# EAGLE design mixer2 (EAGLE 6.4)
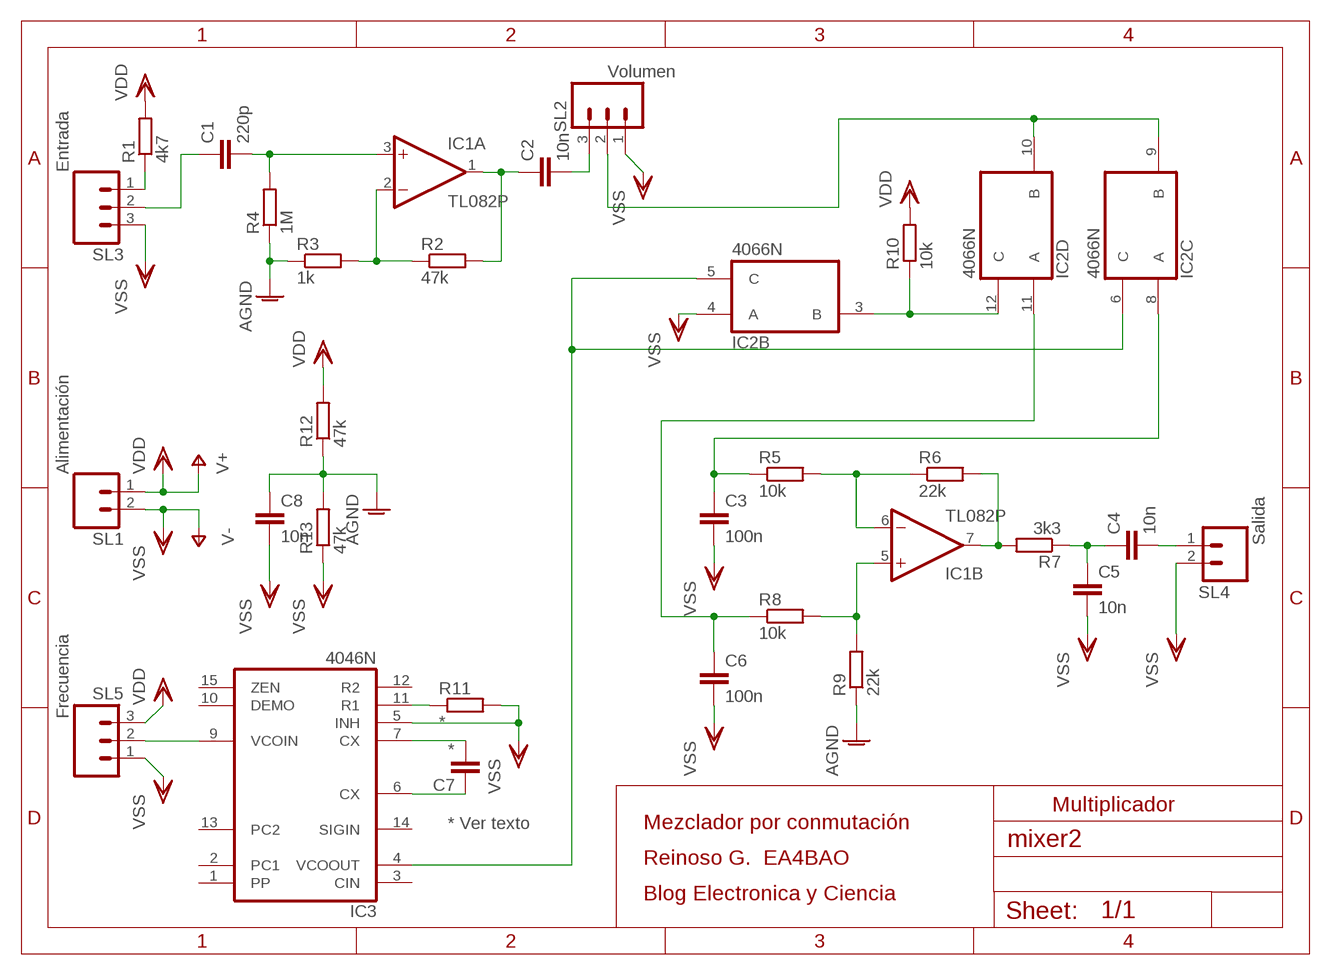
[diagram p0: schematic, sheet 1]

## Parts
C1  220p  C-EU050-035X075  [C050-035X075]
C2  10n  C-EU050-035X075  [C050-035X075]
C3  100n  C-EU050-035X075  [C050-035X075]
C4  10n  C-EU050-035X075  [C050-035X075]
C5  10n  C-EU050-035X075  [C050-035X075]
C6  100n  C-EU050-035X075  [C050-035X075]
C7  *  C-EU050-035X075  [C050-035X075]
C8  10n  C-EU050-035X075  [C050-035X075]
IC1  TL082P  [DIL08]
IC2  4066N  [DIL14]
IC3  4046N  [DIL16]
R1  4k7  R-EU_0207/10  [0207/10]
R2  47k  R-EU_0207/10  [0207/10]
R3  1k  R-EU_0207/10  [0207/10]
R4  1M  R-EU_0207/10  [0207/10]
R5  10k  R-EU_0207/10  [0207/10]
R6  22k  R-EU_0207/10  [0207/10]
R7  3k3  R-EU_0207/10  [0207/10]
R8  10k  R-EU_0207/10  [0207/10]
R9  22k  R-EU_0207/10  [0207/10]
R10  10k  R-EU_0207/10  [0207/10]
R11  *  R-EU_0207/10  [0207/10]
R12  47k  R-EU_0207/10  [0207/10]
R13  47k  R-EU_0207/10  [0207/10]
SL1  Alimentación  M02  [02P]
SL2  Volumen  M03  [03P]
SL3  Entrada  M03  [03P]
SL4  Salida  M02  [02P]
SL5  Frecuencia  M03  [03P]

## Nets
AGND: C8.1 R3.1 R4.1 R9.1 R12.1 R13.2
FLOC: IC2.5(B:C) IC2.6(C:C) IC3.4(VCOOUT)
N$1: R1.1 SL3.1
N$2: C1.1 SL3.2
N$3: C1.2 IC1.3(A:+IN) R4.2
N$4: IC1.6(B:-IN) R5.2 R6.1
N$5: IC1.2(A:-IN) R2.1 R3.2
N$6: C4.1 C5.1 R7.1
N$7: C2.1 IC1.1(A:OUT) R2.2
N$8: C4.2 SL4.1
N$9: C2.2 SL2.3
N$11: IC2.3(B:B) IC2.12(D:C) R10.1
N$12: IC2.9(C:B) IC2.10(D:B) SL2.2
N$13: IC3.9(VCOIN) SL5.2
N$14: IC3.11(R1) R11.1
N$15: C7.1 IC3.6(CX)
N$16: C7.2 IC3.7(CX)
N$18: IC1.7(B:OUT) R6.2 R7.2
N$20: C3.1 IC2.8(C:A) R5.1
N$21: C6.1 IC2.11(D:A) R8.1
N$23: IC1.5(B:+IN) R8.2 R9.2
VDD: R1.2 R10.2 R12.2 SL1.1 SL5.3 ; supply symbol labelled V+
VSS: C3.2 C5.2 C6.2 C8.2 IC2.4(B:A) IC3.5(INH) R11.2 R13.1 SL1.2 SL2.1 SL3.3 SL4.2 SL5.1 ; supply symbol labelled V-
Unconnected: IC2.1(A:A) IC2.2(A:B) IC2.13(A:C) IC3.1(PP) IC3.2(PC1) IC3.3(CIN) IC3.10(DEMO) IC3.12(R2) IC3.13(PC2) IC3.14(SIGIN) IC3.15(ZEN)

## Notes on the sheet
- Multiplicador
- * Ver texto | Mezclador por conmutación
- Reinoso G.  EA4BAO
- Blog Electronica y Ciencia

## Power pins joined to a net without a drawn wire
VDD: IC1.8(P:V+) IC2.14(P:VDD) IC3.16(VDD)
VSS: IC1.4(P:V-) IC2.7(P:VSS) IC3.8(VSS)

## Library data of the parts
C1-C8 = rcl:C-EU: CAPACITOR, European symbol
IC1 = linear:TL082: OP AMP
IC2 = 40xx:4066: Quad bilateral ANALOG SWITCH
IC3 = 40xx:4046: Micropower PLL
R1-R13 = rcl:R-EU_: RESISTOR, European symbol
SL1 SL4 = con-amp-quick:M02: AMP QUICK CONNECTOR; OC_FARNELL: unknown; OC_NEWARK: unknown
SL2 SL3 SL5 = con-amp-quick:M03: AMP QUICK CONNECTOR; OC_FARNELL: unknown; OC_NEWARK: unknown

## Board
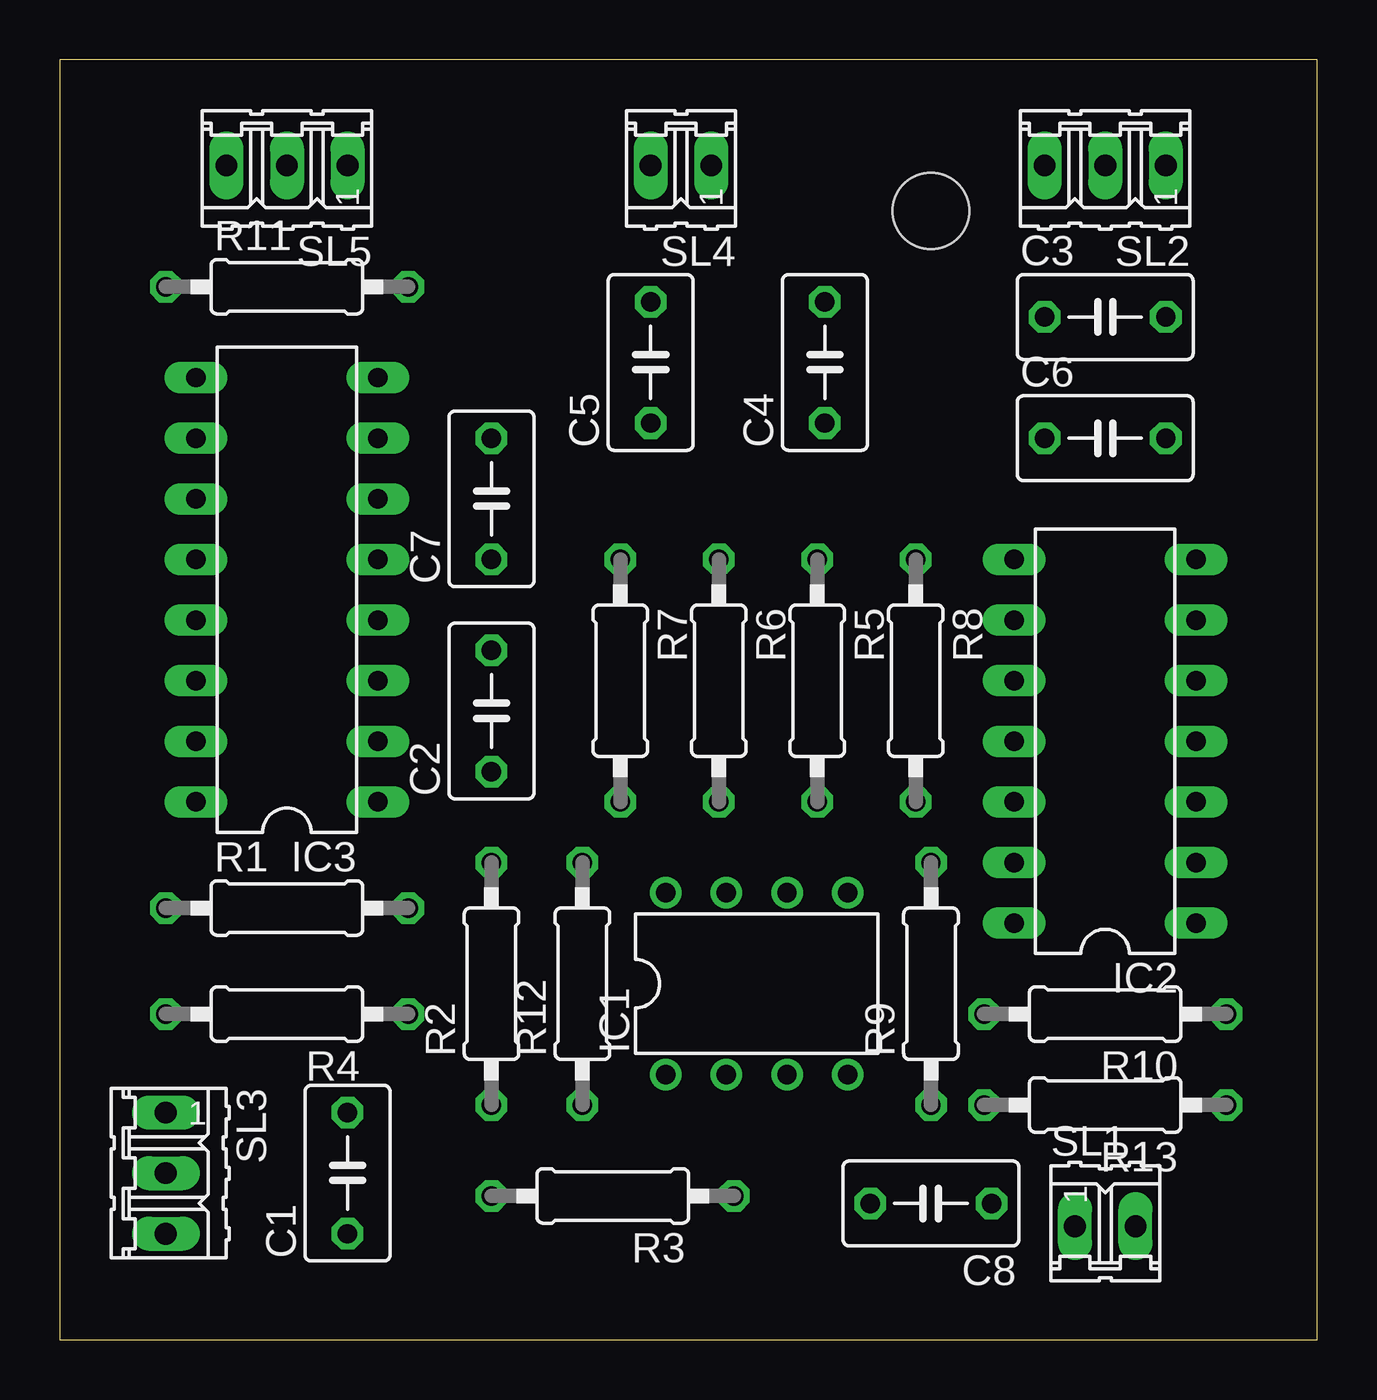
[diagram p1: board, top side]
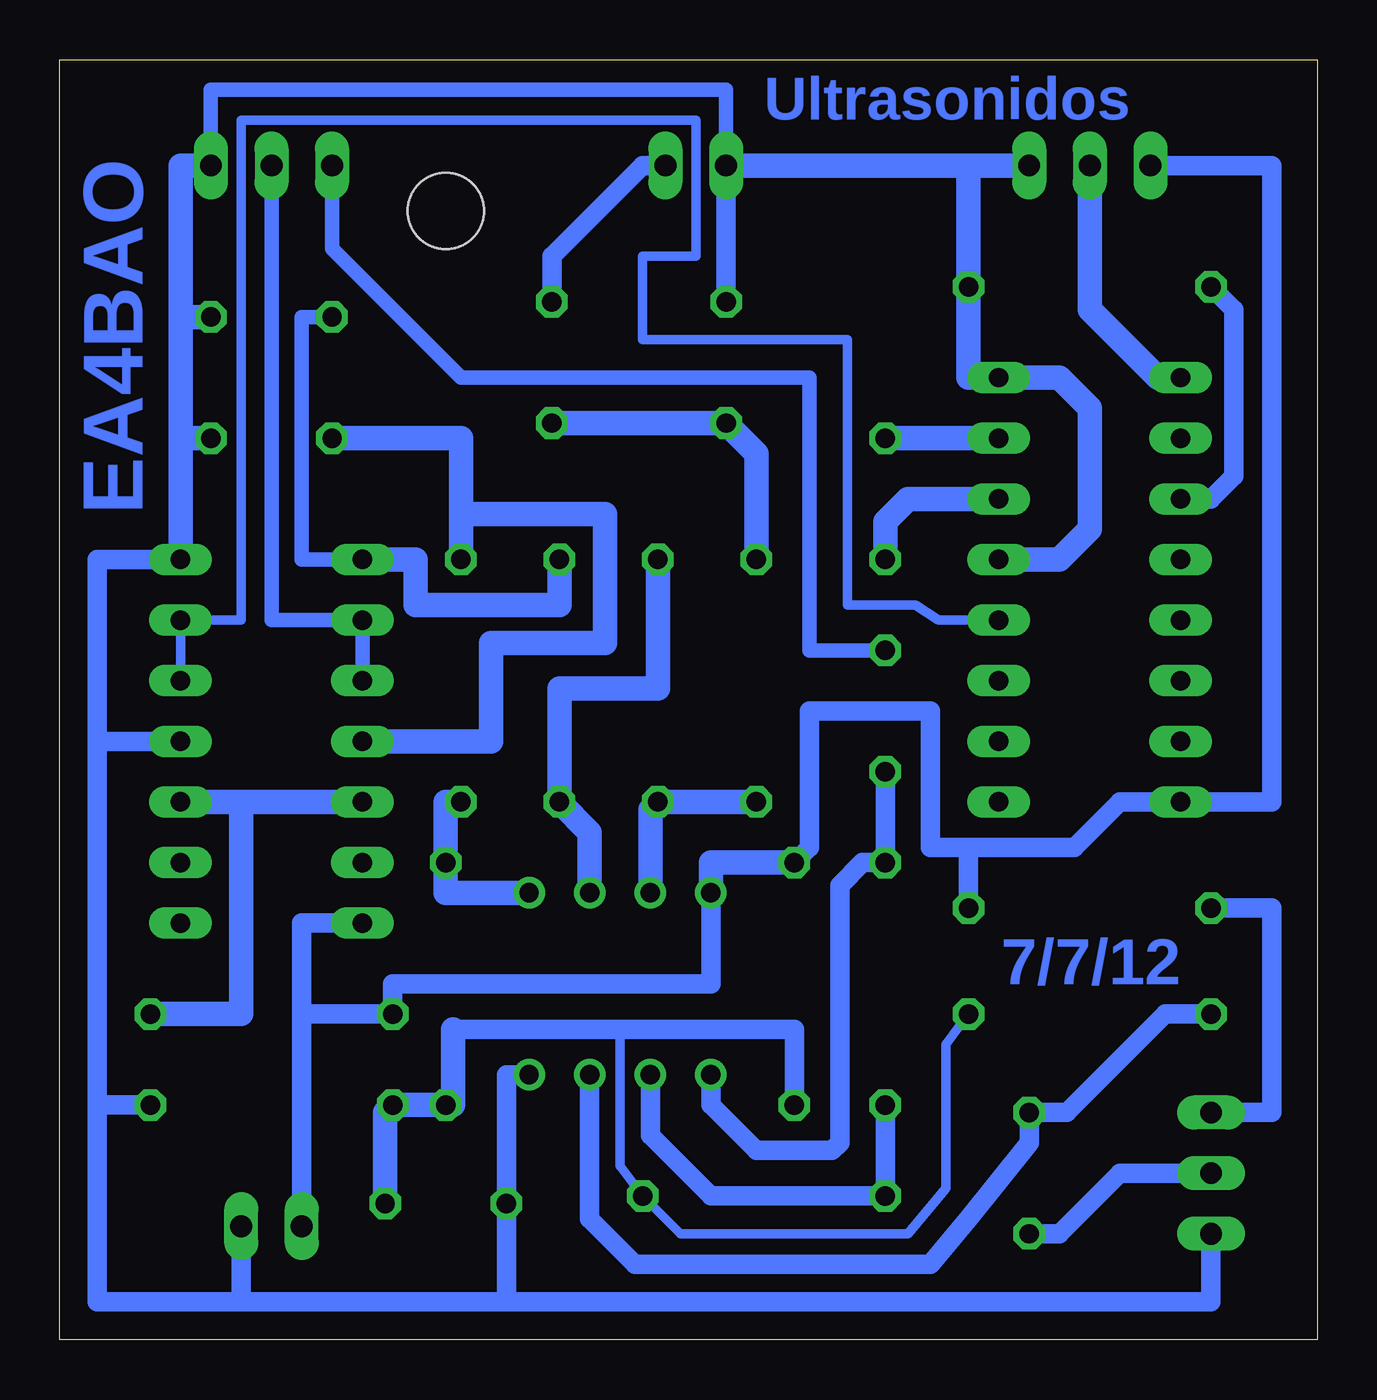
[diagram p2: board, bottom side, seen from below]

Size 52.69 x 53.65 mm. Coordinates in mm from the lower left corner, seen from the top.
Outline: 0,0 52.69,0 52.69,53.65 0,53.65 0,0
Copper layers (1*16): Top 0.035mm / dielectric 1.5mm / Bottom 0.035mm
Design rules "default": minimum track width 10mil, minimum drill 24mil, track to track 8mil, track to pad 8mil, pad to pad 8mil, via to via 8mil, smd to smd 8mil, copper to edge 40mil, drill to drill 8mil, minimum pad ring 10mil, minimum via ring 8mil, stop-mask expansion 4mil, vias tented up to drill 0mil, thermal gap 10mil
Holes 3.2 mm at 36.51,47.31

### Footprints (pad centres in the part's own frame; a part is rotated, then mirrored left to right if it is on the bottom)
C050-035X075 = drill 0.813 octagon: 1 -2.54,0; 2 2.54,0
DIL08 = drill 0.813 pad 1.27: 1 -3.81,-3.81; 2 -1.27,-3.81; 3 1.27,-3.81; 4 3.81,-3.81; 5 3.81,3.81; 6 1.27,3.81; 7 -1.27,3.81; 8 -3.81,3.81
DIL14 = drill 0.813 long: 1 -7.62,-3.81; 2 -5.08,-3.81; 3 -2.54,-3.81; 4 0,-3.81; 5 2.54,-3.81; 6 5.08,-3.81; 7 7.62,-3.81; 8 7.62,3.81; 9 5.08,3.81; 10 2.54,3.81; 11 0,3.81; 12 -2.54,3.81; 13 -5.08,3.81; 14 -7.62,3.81
DIL16 = drill 0.813 long: 1 -8.89,-3.81; 2 -6.35,-3.81; 3 -3.81,-3.81; 4 -1.27,-3.81; 5 1.27,-3.81; 6 3.81,-3.81; 7 6.35,-3.81; 8 8.89,-3.81; 9 8.89,3.81; 10 6.35,3.81; 11 3.81,3.81; 12 1.27,3.81; 13 -1.27,3.81; 14 -3.81,3.81; 15 -6.35,3.81; 16 -8.89,3.81
0207/10 = drill 0.813 octagon: 1 -5.08,0; 2 5.08,0
02P = drill 0.914 long: 1 -1.27,0; 2 1.27,0
03P = drill 0.914 long: 1 -2.54,0; 2 0,0; 3 2.54,0

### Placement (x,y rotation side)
C1  12.06,6.99 90 top
C2  18.1,26.35 90 top
C3  43.81,42.86 0 top
C4  32.07,40.96 90 top
C5  24.77,40.96 90 top
C6  43.81,37.78 0 top
C7  18.1,35.24 90 top
C8  36.51,5.71 180 top
IC1  29.21,14.92 0 top
IC2  43.81,25.08 90 top
IC3  9.53,31.43 90 top
R1  9.53,18.1 0 top
R2  18.1,14.92 90 top
R3  23.18,6.03 180 top
R4  9.53,13.65 180 top
R5  31.75,27.62 270 top
R6  27.62,27.62 270 top
R7  23.5,27.62 270 top
R8  35.88,27.62 270 top
R9  36.51,14.92 90 top
R10  43.81,13.65 180 top
R11  9.53,44.13 0 top
R12  21.91,14.92 90 top
R13  43.81,9.84 180 top
SL1  43.81,4.76 0 top
SL2  43.81,49.21 180 top
SL3  4.45,6.99 270 top
SL4  26.04,49.21 180 top
SL5  9.53,49.21 180 top

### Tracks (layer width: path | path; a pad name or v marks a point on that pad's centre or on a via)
AGND
  Bottom 0.406: 29.21,13.02 29.21,7.3 R3.1 26.67,4.45 17.14,4.45 15.56,6.35 15.56,12.38 R4.1
  Bottom 0.813: R12.1 21.91,13.02 29.21,13.02 36.2,13.02
  Bottom 1.016: 36.2,13.02 36.2,9.84 R9.1 R13.2 39.05,9.52 C8.1
FLOC
  Bottom 0.406: IC2.5 IC2.6 45.09,30.16 45.09,51.12 26.04,51.12 26.04,45.4 28.26,45.4 28.26,41.91 19.68,41.91 19.68,30.8 16.83,30.8 15.88,30.16 IC3.4
N$1
  Bottom 0.813: SL3.1 1.91,9.52 1.91,18.1 R1.1
N$2
  Bottom 0.813: C1.1 10.79,4.45 8.26,6.99 SL3.2
N$3
  Bottom 0.813: R4.2 6.35,13.65 10.48,9.52 C1.2 12.06,8.26 14.61,5.08 16.19,3.17 28.57,3.17 30.48,5.08 IC1.3
N$4
  Bottom 1.016: IC1.6 30.48,21.27 R5.2 31.75,27.31 27.62,27.31 R6.1
N$5
  Bottom 0.813: R2.1 R3.2 25.4,6.03 27.94,8.57 IC1.2
N$6
  Bottom 1.016: C4.1 C5.1 23.5,37.15 R7.1
N$7
  Bottom 0.813: C2.1 R2.2 19.05,20 20,19.05 20,8.26 20.32,7.94 23.5,7.94 25.4,9.84 IC1.1
N$8
  Bottom 0.813: SL4.1 28.26,49.21 32.07,45.4 C4.2
N$9
  Bottom 0.61: C2.2 21.27,28.89 21.27,40.32 35.88,40.32 41.27,45.72 SL2.3
N$11
  Bottom 1.016: 45.09,22.54 IC2.3 | R10.1 45.09,13.65 45.09,22.54 | 45.09,22.54 IC2.12
N$12
  Bottom 0.61: SL2.2 43.81,30.16 IC2.9 IC2.10
N$13
  Bottom 0.813: IC3.9 6.67,40.32
  Bottom 1.016: SL5.2 9.53,43.18 6.67,40.32
N$14
  Bottom 0.813: R11.1 3.49,43.18 3.49,36.19 4.45,35.24 IC3.11
N$15
  Bottom 1.016: IC3.6 17.14,35.24 18.1,34.29 C7.1
N$16
  Bottom 1.016: IC3.7 C7.2
N$18
  Bottom 1.016: R7.2 R6.2 27.94,22.22 IC1.7
N$20
  Bottom 0.61: C3.1 42.55,42.86 42.55,32.7 IC2.8
  Bottom 1.016: IC2.8 37.78,32.7 37.78,30.8 31.75,30.8 R5.1
N$21
  Bottom 1.016: IC2.11 34.61,25.08 34.61,29.21 29.84,29.21 29.84,34.61 35.88,34.61 | 35.88,34.61 R8.1 | C6.1 35.88,37.78 35.88,34.61
N$23
  Bottom 1.016: R8.2 36.51,22.54 R9.2 36.51,18.73 IC1.5
VDD
  Bottom 0.813: IC2.14 42.55,17.46 42.55,13.65 | 42.55,13.65 R10.2 38.73,14.92 25.4,14.92 IC1.8 | IC3.16 4.45,22.54 | IC3.16 1.91,22.54 1.91,49.21 SL5.3 | R12.2 21.27,20.64 21.27,26.35 16.19,26.35 16.19,20.64 14.61,20.64 | 14.61,20.64 R1.2 | IC3.16 8.26,22.54 10.16,20.64 14.61,20.64 | 42.55,13.65 SL1.1
  Bottom 1.016: R12.2 25.4,20 IC1.8
VSS
  Bottom 0.61: SL2.1 46.35,52.39 24.77,52.39 SL4.2
  Bottom 0.813: 33.97,1.59 4.45,1.59 SL3.3 | 33.97,1.59 C8.2 33.97,11.11 IC1.4 | 51.12,9.84 51.12,1.59 45.09,1.59 | 51.12,9.84 R13.1 | 45.09,1.59 SL1.2 | SL4.2 C5.2 | 33.97,1.59 45.09,1.59 | 51.12,9.84 51.12,25.08 | 51.12,25.08 51.12,32.7 IC2.7 | 51.12,25.08 IC2.4
  Bottom 1.016: IC2.7 47.62,37.78 | 47.62,42.86 47.62,49.21 SL2.1 | 47.62,42.86 C3.2 | 47.62,37.78 C6.2 | 14.61,49.21 R11.2 14.61,40.32 IC3.8 10.79,40.32 9.53,39.05 9.53,33.97 10.79,32.7 IC3.5 | 47.62,37.78 47.62,42.86 | 14.61,49.21 SL5.1 | SL4.2 14.61,49.21

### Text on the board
Bottom: Ultrasonidos | EA4BAO | 7/7/12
